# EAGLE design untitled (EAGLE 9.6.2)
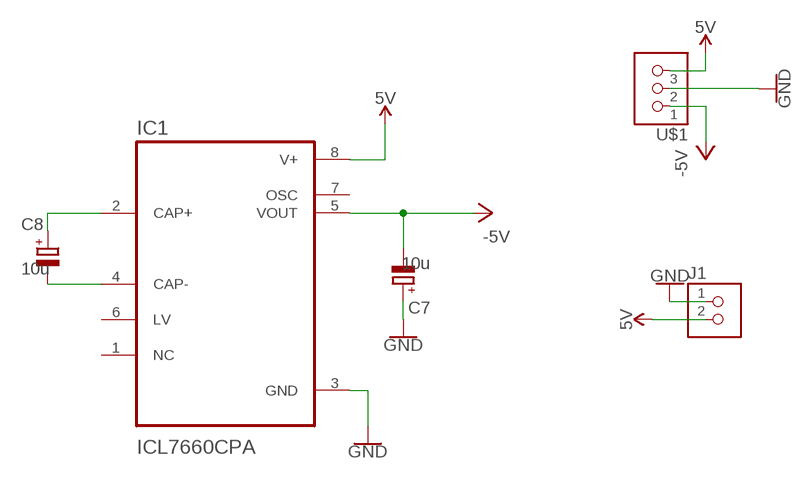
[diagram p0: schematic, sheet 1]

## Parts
C7  10u  CPOL-EU140CLH-0810  [140CLH-0810]
C8  10u  CPOL-EU140CLH-0810  [140CLH-0810]
IC1  ICL7660CPA  [DIP794W47P254L991H457Q8]
J1  CONN_02_TERM-ADAFRUIT  [3.5MMTERM]
U$1  CONN_03_TERM'-FABLAB'  [ED555DS-3DS]

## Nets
5V: IC1.8(V+) J1.2 U$1.3
-5V: C7.- IC1.5(VOUT) U$1.1
GND: C7.+ IC1.3(GND) J1.1 U$1.2
N$18: C8.- IC1.4(CAP-)
N$19: C8.+ IC1.2(CAP+)
Unconnected: IC1.1(NC) IC1.6(LV) IC1.7(OSC)

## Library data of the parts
C7 C8 = rcl:CPOL-EU: POLARIZED CAPACITOR, European symbol; SPICEPREFIX: C
IC1 = ICL7660CPA:ICL7660CPA; AVAILABILITY: Unavailable; DESCRIPTION: Charge Pump Switching Regulator IC Positive or Negative Fixed -Vin, 2Vin 1 Output 45mA 8-DIP (0.300, 7.62mm); DIGIKEY-PURCHASE-URL: https://snapeda.com/shop?store=DigiKey&id=184409; MF: Renesas Electronics; MP: ICL7660CPA; PACKAGE: DIP-8 Intel; PRICE: None
J1 = fab:CONN_02_TERM: 3.5mm terminal block, 2 positions ED555-2DS as found in the fablab inventory.
U$1 = fab:CONN_03_TERM: 3.5mm terminal block, 3 positions ED555-3DS as found in the fablab inventory. Made by Zaerc.

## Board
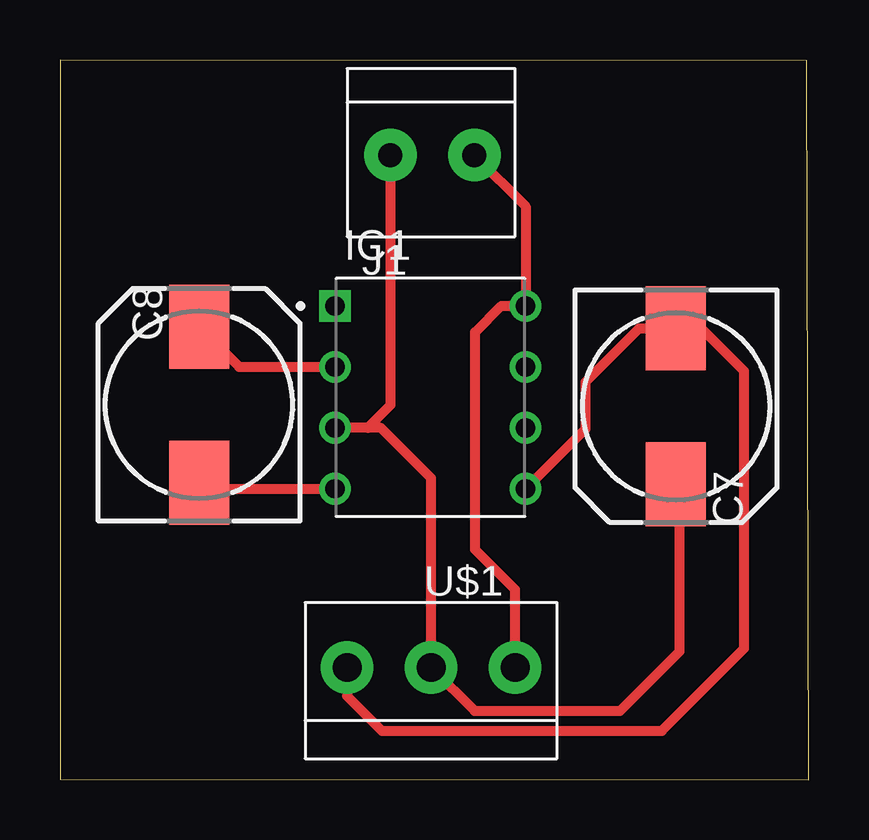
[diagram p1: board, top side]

Size 31.19 x 30 mm. Coordinates in mm from the lower left corner, seen from the top.
Outline: 0,0.03 31.19,0 31.12,29.96 0,30 0,0.03
Copper layers (1*16): Top 0.035mm / dielectric 1.5mm / Bottom 0.035mm
Design rules "default *": minimum track width 16mil, minimum drill 0.4mm, track to track 16mil, track to pad 16mil, pad to pad 16mil, via to via 16mil, smd to smd 16mil, copper to edge 40mil, drill to drill 6mil, minimum pad ring 10mil, minimum via ring 8mil, stop-mask expansion 4mil, vias tented up to drill 0mil, thermal gap 10mil

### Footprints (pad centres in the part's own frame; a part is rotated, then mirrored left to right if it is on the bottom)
140CLH-0810 = smd 3.5 x 2.5: + 3.25,0; - -3.25,0
DIP794W47P254L991H457Q8 = drill 0.81 pad 1.22 square: 1 -3.97,3.81 | drill 0.81 pad 1.22: 2 -3.97,1.27; 3 -3.97,-1.27; 4 -3.97,-3.81; 5 3.97,-3.81; 6 3.97,-1.27; 7 3.97,1.27; 8 3.97,3.81
3.5MMTERM = drill 1 pad 2.184: 1 1.8,0; 2 -1.7,0
ED555DS-3DS = drill 1.2 pad 2.184: 1 -3.5,0; 2 0,0; 3 3.5,0

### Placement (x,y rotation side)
C7  25.67,15.57 270 top
C8  5.8,15.63 90 top
IC1  15.43,15.94 0 top
J1  15.57,26.04 180 top
U$1  15.46,4.69 0 top

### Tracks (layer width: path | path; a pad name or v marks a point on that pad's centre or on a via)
5V
  Top 0.406: U$1.3 18.96,7.93 17.3,9.6 17.3,18.66 18.4,19.75 IC1.8 19.4,23.9 J1.2
-5V
  Top 0.406: IC1.5 21.9,14.63 21.9,16.59 24.13,18.82 C7.- 26.73,18.82 28.51,17.04 28.51,5.48 25.08,2.05 13.41,2.05 11.96,3.5 U$1.1
GND
  Top 0.406: J1.1 13.77,15.61 12.83,14.67 IC1.3 13.37,14.67 15.46,12.58 U$1.2 17.27,2.87 23.33,2.87 25.82,5.36 25.82,12.17 C7.+
N$18
  Top 0.406: C8.- 6.05,12.13 IC1.4
N$19
  Top 0.406: C8.+ 7.47,17.21 IC1.2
